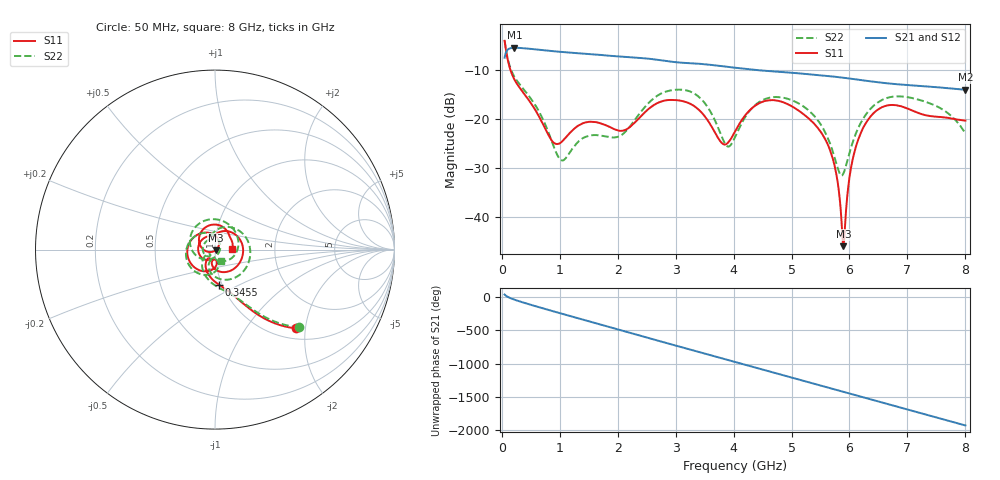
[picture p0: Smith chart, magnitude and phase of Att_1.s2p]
#  HZ  S  DB  R  50.00
! Rohde & Schwarz Vector Network Analyzer
! Rohde-Schwarz,ZNB40-4Port,1311601084101679,3.45
! Created: UTC 4/25/2025, 9:28:53 AM
! freq[Hz]  db:S11  ang:S11  db:S21  ang:S21  db:S12  ang:S12  db:S22  ang:S22
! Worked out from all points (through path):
!   1750 points, 50 MHz to 8 GHz, reference 50 ohm
!   highest |S21| = -5.42 dB at 218.2 MHz (marker M1); lowest = -14.0 dB at 8 GHz (marker M2)
!   group delay of S21, straight-line fit = 668 ps
!   lowest |S11| = -45.9 dB at 5.895 GHz (marker M3), VSWR 1.01, Z = 50.3 - j0.412 ohm
!   |S11| at or under -10 dB: 152 MHz to end of sweep
!   |S22| runs from -31.5 to -3.9 dB; largest |S21 - S12| = 0.00063
!   S11 on the Smith chart (normalised r, x): 50 MHz: 1.22, -1.79; 345.5 MHz: 0.96, -0.39; 8 GHz: 1.21, +0.00
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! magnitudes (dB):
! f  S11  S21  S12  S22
! 50 MHz  -4.0  -7.5  -7.5  -3.9
! 218.2 MHz  -11.9  -5.4  -5.4  -11.3
! 345.5 MHz  -14.2  -5.5  -5.5  -13.4
! 863.6 MHz  -24.4  -6.1  -6.1  -24.5
! 1.014 GHz  -24.8  -6.2  -6.3  -28.2
! 1.377 GHz  -21.0  -6.6  -6.6  -24.0
! 2.05 GHz  -22.4  -7.2  -7.2  -23.4
! 2.7 GHz  -16.6  -7.9  -7.9  -15.1
! 3.305 GHz  -17.2  -8.6  -8.6  -14.6
! 3.818 GHz  -25.1  -9.2  -9.2  -24.2
! 4.027 GHz  -22.5  -9.5  -9.5  -23.6
! 4.577 GHz  -16.2  -10.1  -10.1  -15.8
! 5.35 GHz  -20.4  -10.9  -10.9  -18.8
! 5.709 GHz  -27.9  -11.3  -11.3  -26.5
! 5.795 GHz  -32.8  -11.4  -11.4  -29.9
! 5.895 GHz  -45.9  -11.5  -11.5  -31.1
! 6.014 GHz  -30.8  -11.7  -11.7  -26.3
! 6.15 GHz  -24.2  -11.9  -11.9  -21.8
! 6.382 GHz  -19.2  -12.3  -12.3  -17.6
! 6.677 GHz  -17.1  -12.7  -12.7  -15.6
! 7.491 GHz  -19.5  -13.5  -13.5  -17.3
! 8 GHz  -20.3  -14.0  -14.0  -22.9
